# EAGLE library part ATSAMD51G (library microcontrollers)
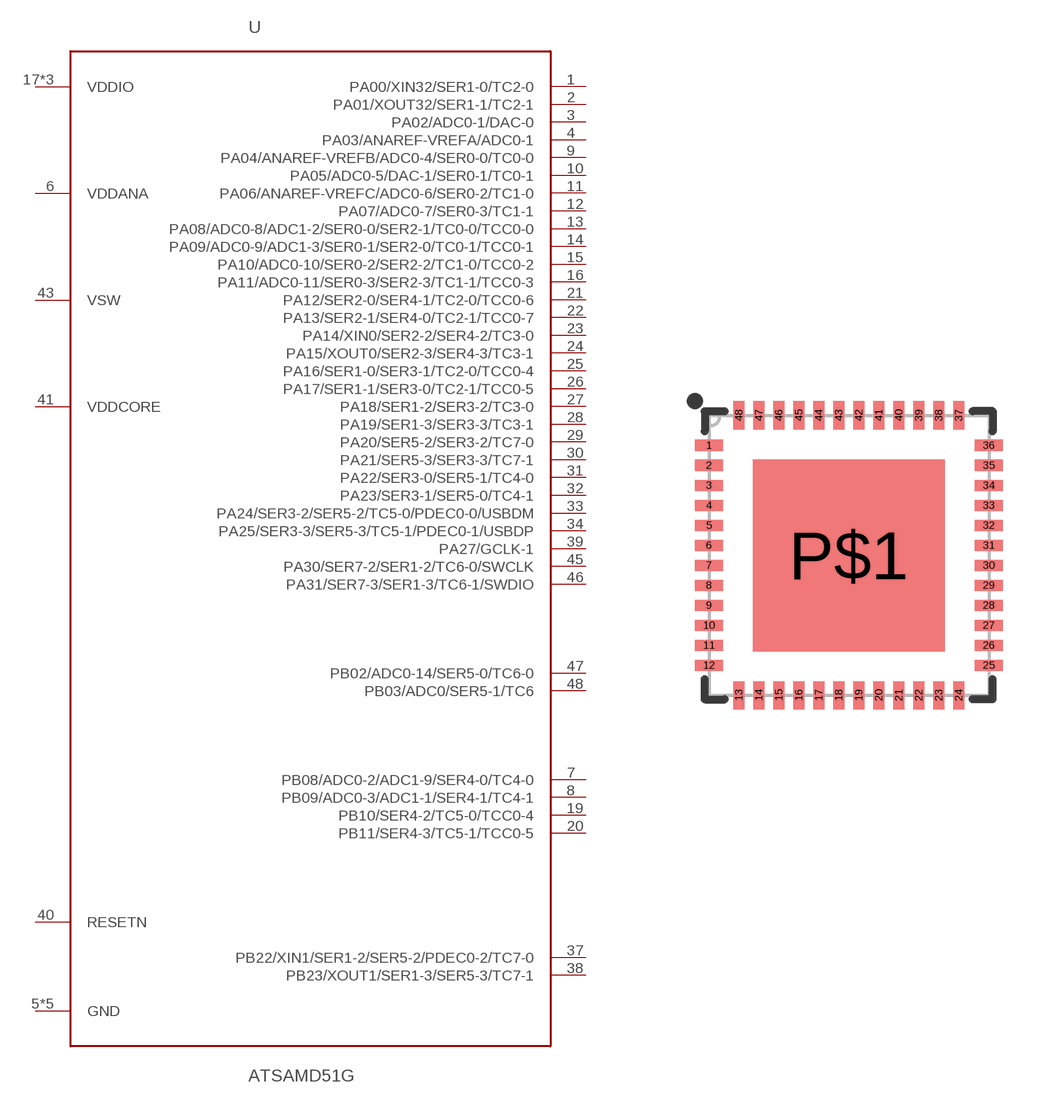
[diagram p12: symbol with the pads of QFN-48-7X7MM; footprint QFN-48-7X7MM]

Designator prefix U

## ATSAMD51GQFN48  [QFN-48-7X7MM]
1  PA00/XIN32/SER1-0/TC2-0
2  PA01/XOUT32/SER1-1/TC2-1
3  PA02/ADC0-1/DAC-0
4  PA03/ANAREF-VREFA/ADC0-1
5  GND
6  VDDANA
7  PB08/ADC0-2/ADC1-9/SER4-0/TC4-0
8  PB09/ADC0-3/ADC1-1/SER4-1/TC4-1
9  PA04/ANAREF-VREFB/ADC0-4/SER0-0/TC0-0
10  PA05/ADC0-5/DAC-1/SER0-1/TC0-1
11  PA06/ANAREF-VREFC/ADC0-6/SER0-2/TC1-0
12  PA07/ADC0-7/SER0-3/TC1-1
13  PA08/ADC0-8/ADC1-2/SER0-0/SER2-1/TC0-0/TCC0-0
14  PA09/ADC0-9/ADC1-3/SER0-1/SER2-0/TC0-1/TCC0-1
15  PA10/ADC0-10/SER0-2/SER2-2/TC1-0/TCC0-2
16  PA11/ADC0-11/SER0-3/SER2-3/TC1-1/TCC0-3
17  VDDIO
18  GND
19  PB10/SER4-2/TC5-0/TCC0-4
20  PB11/SER4-3/TC5-1/TCC0-5
21  PA12/SER2-0/SER4-1/TC2-0/TCC0-6
22  PA13/SER2-1/SER4-0/TC2-1/TCC0-7
23  PA14/XIN0/SER2-2/SER4-2/TC3-0
24  PA15/XOUT0/SER2-3/SER4-3/TC3-1
25  PA16/SER1-0/SER3-1/TC2-0/TCC0-4
26  PA17/SER1-1/SER3-0/TC2-1/TCC0-5
27  PA18/SER1-2/SER3-2/TC3-0
28  PA19/SER1-3/SER3-3/TC3-1
29  PA20/SER5-2/SER3-2/TC7-0
30  PA21/SER5-3/SER3-3/TC7-1
31  PA22/SER3-0/SER5-1/TC4-0
32  PA23/SER3-1/SER5-0/TC4-1
33  PA24/SER3-2/SER5-2/TC5-0/PDEC0-0/USBDM
34  PA25/SER3-3/SER5-3/TC5-1/PDEC0-1/USBDP
35  GND
36  VDDIO
37  PB22/XIN1/SER1-2/SER5-2/PDEC0-2/TC7-0
38  PB23/XOUT1/SER1-3/SER5-3/TC7-1
39  PA27/GCLK-1
40  RESETN
41  VDDCORE
42  GND
43  VSW
44  VDDIO
45  PA30/SER7-2/SER1-2/TC6-0/SWCLK
46  PA31/SER7-3/SER1-3/TC6-1/SWDIO
47  PB02/ADC0-14/SER5-0/TC6-0
48  PB03/ADC0/SER5-1/TC6
P$1  GND

## Footprint QFN-48-7X7MM (pad centres in mm)
64-pin QFN 9x9mm, 0.5mm pitch Package used by ATmega128RFA1 Example Datasheet
smd 0.7 x 0.275: 1 -3.5,2.75; 2 -3.5,2.25; 3 -3.5,1.75; 4 -3.5,1.25; 5 -3.5,0.75; 6 -3.5,0.25; 7 -3.5,-0.25; 8 -3.5,-0.75; 9 -3.5,-1.25; 10 -3.5,-1.75; 11 -3.5,-2.25; 12 -3.5,-2.75; 25 3.5,-2.75; 26 3.5,-2.25; 27 3.5,-1.75; 28 3.5,-1.25; 29 3.5,-0.75; 30 3.5,-0.25; 31 3.5,0.25; 32 3.5,0.75; 33 3.5,1.25; 34 3.5,1.75; 35 3.5,2.25; 36 3.5,2.75
smd 0.275 x 0.7: 13 -2.75,-3.5; 14 -2.25,-3.5; 15 -1.75,-3.5; 16 -1.25,-3.5; 17 -0.75,-3.5; 18 -0.25,-3.5; 19 0.25,-3.5; 20 0.75,-3.5; 21 1.25,-3.5; 22 1.75,-3.5; 23 2.25,-3.5; 24 2.75,-3.5; 37 2.75,3.5; 38 2.25,3.5; 39 1.75,3.5; 40 1.25,3.5; 41 0.75,3.5; 42 0.25,3.5; 43 -0.25,3.5; 44 -0.75,3.5; 45 -1.25,3.5; 46 -1.75,3.5; 47 -2.25,3.5; 48 -2.75,3.5
smd 4.8 x 4.8: P$1 0,0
